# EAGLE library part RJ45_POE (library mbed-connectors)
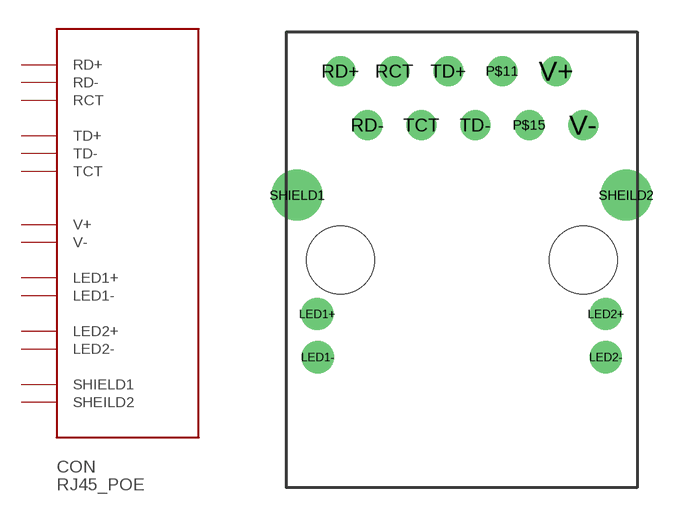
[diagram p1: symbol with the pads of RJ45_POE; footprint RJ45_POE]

Designator prefix CON

## RJ45_POE  [RJ45_POE]
LED1+  LED1+
LED1-  LED1-
LED2+  LED2+
LED2-  LED2-
RCT  RCT
RD+  RD+
RD-  RD-
SHEILD2  SHEILD2
SHIELD1  SHIELD1
TCT  TCT
TD+  TD+
TD-  TD-
V+  V+
V-  V-

## Footprint RJ45_POE (pad centres in mm)
Tyco 1-6605834-1 RJ45 Jack PoE
drill 1.016: LED1+ -6.807,-2.54; LED1- -6.782,-4.572; LED2+ 6.782,-2.54; LED2- 6.782,-4.572
drill 0.9: P$11 1.905,8.89; P$15 3.175,6.35; RCT -3.175,8.89; RD+ -5.715,8.89; RD- -4.445,6.35; TCT -1.905,6.35; TD+ -0.635,8.89; TD- 0.635,6.35; V+ 4.445,8.89; V- 5.715,6.35
drill 1.6: SHEILD2 7.747,3.048; SHIELD1 -7.747,3.048
hole 3.2 at -5.715,0
hole 3.2 at 5.715,0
